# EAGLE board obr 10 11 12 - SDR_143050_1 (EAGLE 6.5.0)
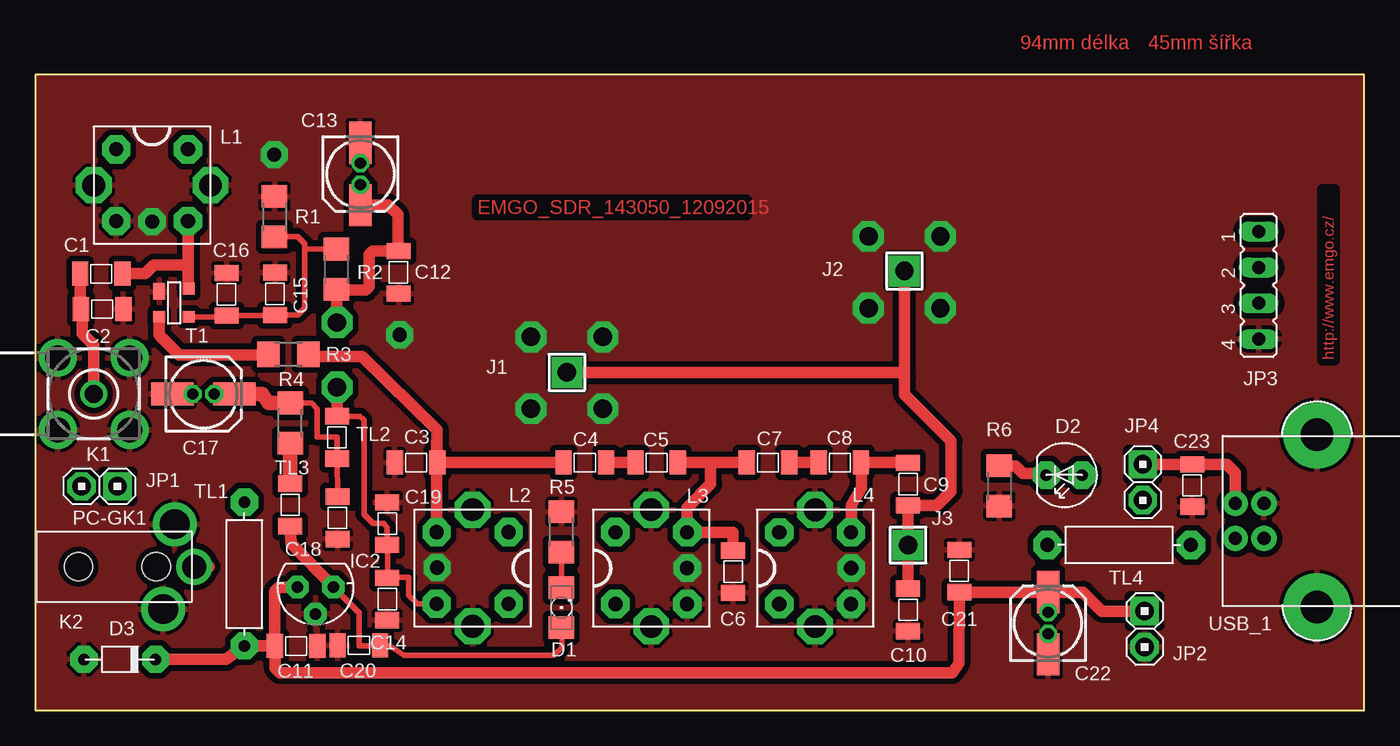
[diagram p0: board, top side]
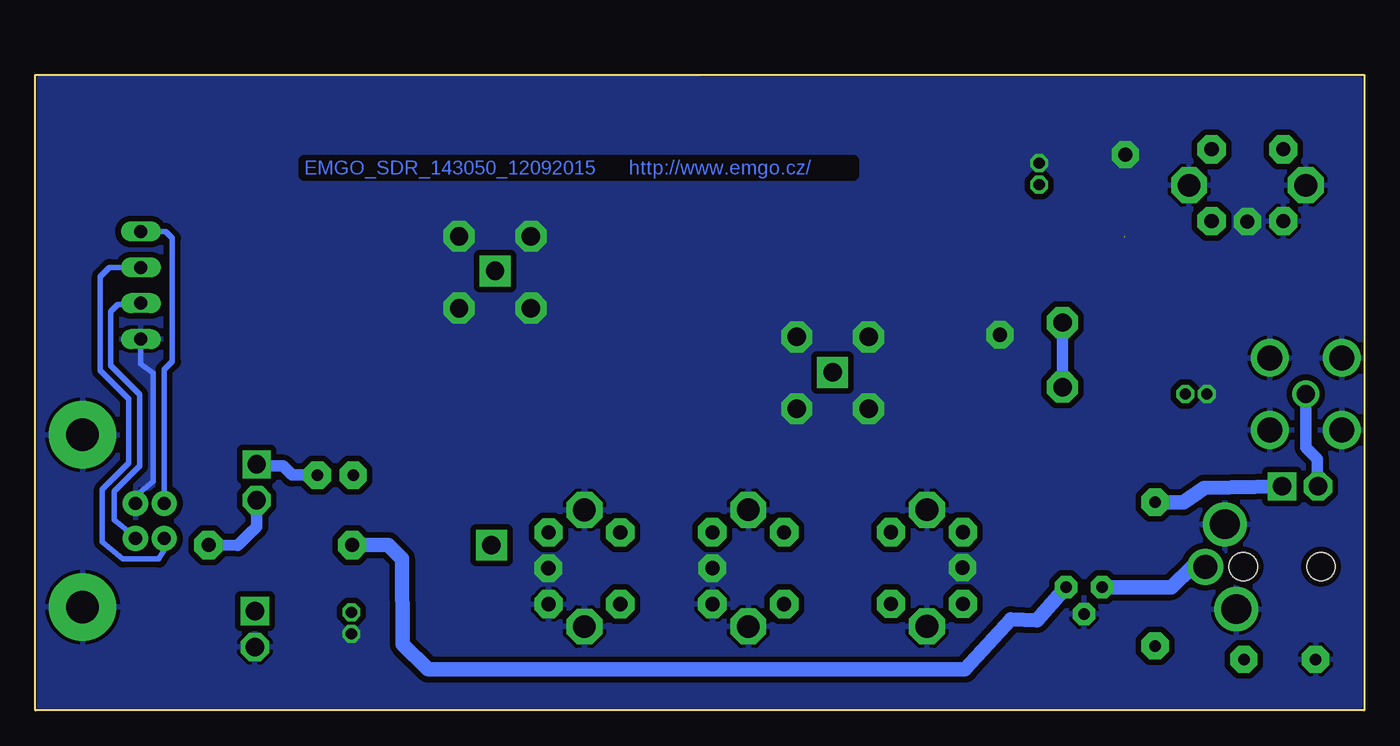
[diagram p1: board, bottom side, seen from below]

Size 93.98 x 44.96 mm. Coordinates in mm from the lower left corner, seen from the top.
Outline: 0,0 93.98,0 93.98,44.96 0,44.96 0,0
Copper layers (1*16): Top 0.035mm / dielectric 1.5mm / Bottom 0.035mm
Design rules "default": minimum track width 10mil, minimum drill 24mil, track to track 8mil, track to pad 8mil, pad to pad 8mil, via to via 8mil, smd to smd 8mil, copper to edge 0mil, drill to drill 8mil, minimum pad ring 10mil, minimum via ring 8mil, stop-mask expansion 0mil, vias tented up to drill 0mil, thermal gap 10mil

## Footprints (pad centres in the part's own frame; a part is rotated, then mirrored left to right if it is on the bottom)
SMD-1206 = smd 1.15 x 1.7: 1 -1.5,0; 2 1.5,0
153CLV-0505 = smd 3 x 1.6: + 2.2,0; - -2.2,0
1206 = smd 1.6 x 1.803: A -1.422,0; C 1.422,0
LED = drill 0.813 pad 1.93 octagon: A 0,0; K 2.54,0
D-5 = drill 0.813 pad 1.93 octagon: 1 -2.54,0; 2 2.54,0
78LXX = drill 0.813 pad 1.6 octagon: GND 0,1.905; IN 1.27,0; OUT -1.27,0
PAD-01 = drill 1.3 pad 2.184 square: 1 0,0
PINH-2 = drill 1.3 pad 2 square: 1 0,0 | drill 1.3 pad 2 octagon: 2 2.54,0
JP4 = drill 0.914 long: 1 -3.81,0; 2 -1.27,0; 3 1.27,0; 4 3.81,0
BU-SMA-H = drill 1.27: 1 0,0 | drill 1.778: 2 -2.55,2.55; 3 2.55,2.55; 4 2.55,-2.55; 5 -2.55,-2.55
PC-GK = drill 1.7 pad 2.54: P$1 8.2,0 | drill 2.1 pad 3: P$2 6,-3; P$3 6.8,3 | hole 2: 5.5,0; 0,0
L-VF50 = drill 1 pad 2 octagon: 1 -2.54,-2.54; 2 2.54,-2.54; 3 2.54,2.54; 4 -2.54,2.54 | drill 1.6 pad 2.54 octagon: 5 -4.128,0; 6 4.128,0
R1206 = smd 1.6 x 1.803: 1 -1.422,0; 2 1.422,0
SOT-143 = smd 1.194 x 0.838: 1 -0.813,-1.041 | smd 0.838 x 0.838: 2 0.991,-1.041; 3 0.991,1.041; 4 -1.016,1.041
L-10@2 = drill 0.813 pad 1.93 octagon: 1 -5.08,0; 2 5.08,0
L-10 = drill 1 pad 2 octagon: 1 -5.08,0; 2 5.08,0
USB1X90B = drill 0.92 pad 1.778: 1 -1.016,1.245; 2 -1.016,-1.245; 3 1.016,-1.245; 4 1.016,1.245 | drill 2.3 pad 4.778: P$3 4.75,-6.096; P$4 4.75,6.096

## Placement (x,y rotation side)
C1  5.6pF  [SMD-1206]  4.67,30.89 0 top
C2  33pF  [SMD-1206]  4.73,28.38 180 top
C3  8.2pF  [SMD-1206]  26.92,17.53 0 top
C4  1pF  [SMD-1206]  38.86,17.53 180 top
C5  1pF  [SMD-1206]  43.94,17.53 180 top
C6  6.8pF  [SMD-1206]  49.35,9.8 90 top
C7  1pF  [SMD-1206]  51.82,17.53 180 top
C8  1pF  [SMD-1206]  56.9,17.53 180 top
C9  6.8pF  [SMD-1206]  61.72,16 90 top
C10  33pF  [SMD-1206]  61.72,7.11 90 top
C11  100nF  [SMD-1206]  18.44,4.55 0 top
C12  100nF  [SMD-1206]  25.69,30.99 90 top
C13  10M  [153CLV-0505]  22.99,37.94 270 top
C14  100nF  [SMD-1206]  24.89,7.87 90 top
C15  1nF  [SMD-1206]  16.95,29.46 270 top
C16  100nF  [SMD-1206]  13.53,29.43 270 top
C17  10M  [153CLV-0505]  11.89,22.38 0 top
C18  100nF  [SMD-1206]  21.37,13.61 270 top
C19  1nF  [SMD-1206]  24.89,13.21 270 top
C20  100nF  [SMD-1206]  22.89,4.6 180 top
C21  100nF  [SMD-1206]  65.34,9.86 90 top
C22  10M  [153CLV-0505]  71.63,6.16 90 top
C23  100nF  [SMD-1206]  81.81,15.9 90 top
D1  LED  [1206]  37.21,7.26 90 top
D2  LED  [LED]  74.04,16.64 180 top
D3  protect  [D-5]  5.97,3.61 0 top
IC2  78L05  [78LXX]  19.81,8.71 180 top
J1  [PAD-01]  37.59,23.91 0 top
J2  [PAD-01]  61.47,31.08 0 top
J3  [PAD-01]  61.72,11.68 0 top
JP1  [PINH-2]  5.81,15.84 180 top
JP2  UCC-GND  [PINH-2]  78.45,7.02 270 top
JP3  [JP4]  86.52,30.07 270 top
JP4  USB-UCC  [PINH-2]  78.33,17.4 270 top
K1  [BU-SMA-H]  4.13,22.38 180 top
K2  PC-GK1  [PC-GK]  3.05,10.16 0 top
L1  2.75z  [L-VF50]  8.26,37.15 0 top
L2  2.75z  [L-VF50]  30.92,10.06 270 top
L3  2.75z  [L-VF50]  43.56,10.06 90 top
L4  2.75z  [L-VF50]  55.15,10.05 90 top
R1  100K  [R1206]  16.92,34.92 90 top
R2  100K  [R1206]  21.3,31.21 270 top
R3  47R  [R1206]  17.89,25.18 0 top
R4  2R2  [R1206]  18.03,20.32 270 top
R5  1K  [R1206]  37.21,12.62 270 top
R6  1K  [R1206]  68.17,15.88 90 top
T1  BF998  [SOT-143]  9.81,28.83 270 top
TL1  10uH  [L-10@2]  14.78,9.64 270 top
TL2  10uH  [SMD-1206]  21.34,19.3 270 top
TL3  10uH  [SMD-1206]  18.02,14.54 270 top
TL4  10uH  [L-10]  76.65,11.69 180 top
USB_1  [USB1X90B]  85.88,13.4 0 top

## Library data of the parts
C1-C12 C14-C16 C18-C21 C23 D2 D3 J1-J3 JP1 JP2 JP4 L1-L4 TL1-TL4 = M
C13 C17 C22 = rcl
D1 = led
IC2 = V-REG
JP3 = jumper
K1 = con-coax; OC_FARNELL: unknown; OC_NEWARK: unknown
K2 = CON-POWER
R1-R6 = rcl-2
T1 = TRANS-M
USB_1 = EMGO_BNC

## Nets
GND: C2.1 C3.1 C6.1 C10.1 C11.2 C12.1 C13.- C14.1 C15.1 C16.1 C17.- C18.2 C19.1 C20.2 C21.2 C22.- C23.1 D3.1 IC2.GND JP2.2 JP3.4 K1.2 K1.3 K1.4 K1.5 K2.P$2 K2.P$3 L1.1 L1.5 L1.6 L2.5 L2.6 L3.1 L3.5 L3.6 L4.1 L4.5 L4.6 R1.2 R5.1 R6.1 T1.1 USB_1.4 USB_1.P$3 USB_1.P$4
N$1: C23.2 D2.A JP3.1 JP4.1 USB_1.1
N$2: JP4.2 TL4.1
N$3: JP3.2 USB_1.2
N$4: JP3.3 USB_1.3
N$5: C7.1 C8.2
N$6: R3.1 T1.2
N$7: C1.1 C2.2 JP1.2 K1.1
N$8: C5.1 C6.2 C7.2 L3.2
N$9: C4.1 C5.2
N$10: D1.C R5.2
N$11: C20.1 D1.A IC2.OUT TL3.2 TL4.2
N$12: R4.2 TL3.1
N$13: C17.+ C18.1 R4.1 TL2.2
N$18: JP1.1 TL1.1
N$21: D2.K R6.2
N$26: C11.1 C21.1 C22.+ D3.2 IC2.IN JP2.1 K2.P$1 TL1.2
N$27: C9.1 C10.2 J1.1 J2.1 J3.1
N$29: C8.1 C9.2 L4.2
N$36: C3.2 C4.2 L2.1 R3.2
N$38: C12.2 C13.+ C14.2 C19.2 L2.2 R2.2 TL2.1
N$44: C1.2 L1.2 T1.4
N$50: C15.2 C16.2 R1.1 R2.1 T1.3

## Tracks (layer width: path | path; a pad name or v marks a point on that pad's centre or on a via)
GND  (via drill 0.8 pad 1.27, 1 pad 1.93, 1.3 pad 2.18)
  Bottom 0.406: USB_1.4 86.9,15.18 85.63,16.19 85.63,23.88 86.52,24.51 JP3.4
  other vias: 28.42,10.1 57.7,10.06 8.26,34.58 16.89,39.31 25.77,26.57 46.1,10.06 11.13,22.38 71.63,5.41 22.99,38.71 35.05,26.42 35.05,21.34 40.13,26.42 40.13,21.34 58.93,33.53 58.93,28.45 64.01,33.53 64.01,28.45
  pour Bottom (isolate 0.406): 0.32,0.32 93.66,0.32 93.66,44.74 0.32,44.64
  pour Top (isolate 0.406): 0.32,44.77 93.73,44.77 93.73,0.25 0.25,0.25 0.25,44.7
N$1
  Top 0.813: JP4.1 C23.2 84.26,17.4 84.87,16.79 USB_1.1
  Bottom 0.406: USB_1.1 84.87,24.1 84.3,24.67 84.3,33.4 84.77,33.88 JP3.1
  Bottom 0.813: D2.A 75.82,16.64 76.45,17.27 78.2,17.27 JP4.1
N$2
  Bottom 0.813: JP4.2 78.33,12.99 78.61,12.7 78.64,12.7 79.65,11.68 TL4.1
N$3
  Bottom 0.406: USB_1.2 84.87,11.34 85.25,10.7 87.79,10.7 89.25,11.91 89.25,15.62 87.38,17.49 87.38,22.04 89.38,24.04 89.38,30.7 88.74,31.34 JP3.2
N$4
  Bottom 0.406: USB_1.3 86.9,12.22 88.39,13.46 88.39,15.49 86.61,17.27 86.61,22.35 88.65,24.38 88.65,28.19 88.14,28.7 86.61,28.7 JP3.3
N$5
  Top 0.813: C7.1 C8.2
N$6
  Top 0.813: R3.1 15.63,25.15 10.16,25.15 8.77,26.54 T1.2
N$7
  Top 0.813: C1.1 3.17,28.45 C2.2 3.3,28.31 3.3,26.67 4.13,25.84 K1.1
  Bottom 0.813: K1.1 4.13,18.61 3.3,17.78 3.3,15.88 JP1.2
N$8
  Top 0.813: C5.1 47.75,17.53 | 47.75,17.53 C7.2 | 47.75,17.53 47.75,16 46.1,14.33 L3.2 49.35,12.6 C6.2
N$9
  Top 0.813: C4.1 C5.2
N$10
  Top 0.406: D1.C R5.2
N$11
  Top 0.406: D1.A 37.24,4.45 36.65,3.89 26.09,3.89 25.04,4.57 22.89,4.57 | 22.89,4.57 C20.1 | 22.89,4.57 22.89,6.91 IC2.OUT
  Top 0.813: IC2.OUT 18.09,11.81 TL3.2
  Bottom 1.016: TL4.2 69.02,11.69 68.05,10.72 68,4.67 66.19,2.9 28.22,2.9 24.97,6.45 23.14,6.38 IC2.OUT
N$12
  Top 1.016: TL3.1 R4.2
N$13
  Top 0.406: C18.1 TL2.2 21.34,19.33 19.94,19.33 19.94,21.31 19.56,21.74 R4.1
  Top 1.016: R4.1 16.48,21.74 16.05,22.38 C17.+
N$18
  Bottom 1.016: JP1.1 11.3,15.75 12.8,14.71 TL1.1
N$21
  Top 0.813: R6.2 69.32,17.3 69.85,16.76 71.37,16.76 D2.K
N$26
  Top 0.813: K2.P$1 12.27,10.16 12.29,10.13 | JP2.1 75.44,7.01 74.09,8.36 C22.+ C21.1 65.32,3.31 64.85,2.67 17.27,2.67 16.97,2.97 16.97,4.52 C11.1 | D3.2 13.5,3.61 TL1.2 16.93,4.56 C11.1 | C11.1 16.94,8.43 17.22,8.71 IC2.IN
  Bottom 0.813: 11.27,10.19 K2.P$1
  Bottom 1.016: IC2.IN 13.64,8.71 12.14,10.16 K2.P$1
N$27
  Top 0.813: C10.2 J3.1 C9.1 63.78,14.5 64.77,15.49 64.77,19.05 61.47,22.35 61.47,23.62 | 61.47,23.62 J2.1 | J1.1 61.18,23.91 61.47,23.62
N$28  (via drill 0.8 pad 1.27)
  other vias: 22.99,37.19
N$29
  Top 0.813: C9.2 61.7,17.53 C8.1 58.42,17.5 58.42,15.75 57.72,14.54 L4.2
N$30  (via drill 0.8 pad 1.27)
  other vias: 71.63,6.93
N$33  (via drill 0.8 pad 1.27)
  other vias: 12.65,22.38
N$36
  Top 0.813: C3.2 28.38,19.01 L2.1 | R3.2 20.06,25.04 23.11,25.04 28.42,19.84 C3.2 | C3.2 C4.2
N$38  (via drill 1.3 pad 2.18)
  Top 0.406: L2.2 27.02,7.53 26.42,8.13 26.42,9.4 24.92,9.4 | 24.92,9.4 C14.2 | 24.92,9.4 24.92,11.68 C19.2 24.89,12.95 24.64,13.21 23.88,13.21 23.24,13.87 23.24,20.55 22.99,20.8 TL2.1
  Top 0.813: v21.34,27.43 21.3,27.46 R2.2 21.38,29.72 23.37,29.72 23.62,29.97 23.62,32.26 23.85,32.49 C12.2 25.65,32.52 25.65,35.05 24.96,35.74 C13.+ | v21.34,22.86 TL2.1
  Bottom 0.813: v21.34,27.43 v21.34,22.86
N$44
  Top 0.813: L1.2 10.79,31.5 | 10.79,31.5 10.79,29.9 T1.4 | C1.2 7.78,30.89 8.38,31.5 10.79,31.5
N$50  (1 unrouted)
  Top 0.406: T1.3 13.43,27.84 C16.2 16.92,27.93 C15.2 18.57,27.96 19.05,28.45 19.05,32.51 | 19.05,32.51 19.05,33.02 18.54,33.53 16.95,33.53 | R2.1 19.17,32.63 19.05,32.51

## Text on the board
Top: 94mm délka | 45mm šířka | EMGO_SDR_143050_12092015 | http://www.emgo.cz/
Bottom: EMGO_SDR_143050_12092015 http://www.emgo.cz/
